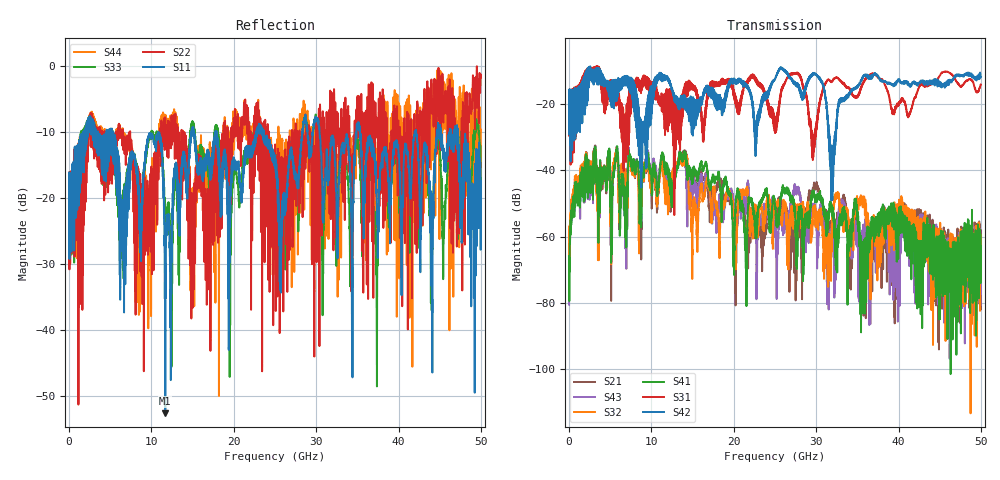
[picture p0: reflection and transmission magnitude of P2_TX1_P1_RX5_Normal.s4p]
!Keysight Technologies,N5225B,MY57041031,A.13.20.10
!Date: Friday, May 31, 2019 11:21:24
!Correction: S11(Full 4 Port(1,2,3,4))
!S12(Full 4 Port(1,2,3,4))
!S13(Full 4 Port(1,2,3,4))
!S14(Full 4 Port(1,2,3,4))
!S21(Full 4 Port(1,2,3,4))
!S22(Full 4 Port(1,2,3,4))
!S23(Full 4 Port(1,2,3,4))
!S24(Full 4 Port(1,2,3,4))
!S31(Full 4 Port(1,2,3,4))
!S32(Full 4 Port(1,2,3,4))
!S33(Full 4 Port(1,2,3,4))
!S34(Full 4 Port(1,2,3,4))
!S41(Full 4 Port(1,2,3,4))
!S42(Full 4 Port(1,2,3,4))
!S43(Full 4 Port(1,2,3,4))
!S44(Full 4 Port(1,2,3,4))
!S4P File: Measurements: <S11,S12,S13,S14>,
!<S21,S22,S23,S24>,
!<S31,S32,S33,S34>,
!<S41,S42,S43,S44>:
# Hz S  dB  R 50.0
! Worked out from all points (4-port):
!   5000 points, 10 MHz to 50 GHz, reference 50 ohm
!   strongest paths, dB at 10 MHz, 12.51 GHz, 25.01 GHz, 37.51 GHz, 50 GHz:
!     S42: -19.5, -15.4, -12.7, -11.6, -11.9
!     S31: -19.6, -17.3, -28.8, -12.1, -14.3
!     S41: -65.9, -49.3, -51.8, -57.1, -69.2
!     S32: -57.0, -42.1, -49.0, -58.6, -65.7
!     S43: -80.5, -46.5, -58.7, -60.9, -61.2
!     S21: -59.9, -44.0, -51.6, -62.4, -59.8
!   lowest |S11| = -52.6 dB at 11.69 GHz (marker M1), VSWR 1.00, Z = 49.8 - j0.0995 ohm
!   |S11| at or under -10 dB: 5.36 GHz to 10.81 GHz (5.45 GHz wide, 67.4 % of centre); 17.89 GHz to 22.7 GHz (4.805 GHz wide, 23.7 % of centre); 35.31 GHz to 41.96 GHz (6.644 GHz wide, 17.2 % of centre)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
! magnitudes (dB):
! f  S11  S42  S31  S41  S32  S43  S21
! 10 MHz  -19.6  -19.5  -19.6  -65.9  -57.0  -80.5  -59.9
! 2.11 GHz  -11.9  -15.5  -14.1  -35.4  -35.1  -35.9  -34.6
! 11.69 GHz  -52.6  -11.9  -22.8  -38.5  -44.0  -39.3  -41.7
! 29.88 GHz  -8.3  -11.0  -29.6  -48.6  -52.5  -51.2  -44.9
! 31.94 GHz  -11.2  -35.8  -13.3  -51.1  -60.4  -56.5  -58.4
! 35.81 GHz  -20.0  -11.4  -13.5  -63.3  -49.0  -60.6  -65.8
! 50 GHz  -17.4  -11.9  -14.3  -69.2  -65.7  -61.2  -59.8
